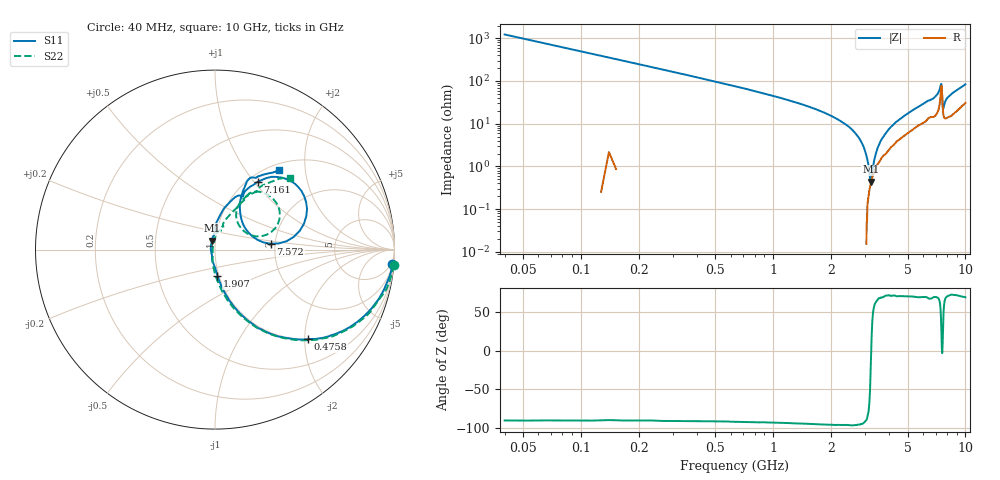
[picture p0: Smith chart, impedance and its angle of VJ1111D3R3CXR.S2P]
! VJ1111D3R3CXR
! DATE 03/04/2022  13:50
! CAPACITORS MOUNTED IN SERIES ON 25 MIL THICK MICROSTRIP SUBSTRATE
# GHz  S  MA  R  50.00
!  FREQ  S11M  S11A  S21M  S21A  S12M  S12A  S22M  S22A
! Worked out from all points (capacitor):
!   801 points, 40 MHz to 10 GHz, reference 50 ohm
!   read as one part in series: C = 3.19 pF near 89.8 MHz
!   lowest |Z| = 436 mohm at 3.215 GHz (marker M1)
!   series resonance near 3.233 GHz, so ESL is about 760 pH
!   S11 on the Smith chart (normalised r, x): 40 MHz: 3, -25; 475.8 MHz: 1.00, -2.06; 1.907 GHz: 0.98, -0.29; 7.161 GHz: 1.11, +1.04; 7.572 GHz: 1.89, +0.14; 10 GHz: 1.11, +1.46
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0.04  0.9893 -4.5  0.08065 85.4  0.08104 85.2  0.9995 -4.9
0.20185  0.9245 -21.8  0.3788 68.4  0.379 68.8  0.9318 -21.9
0.47575  0.7181 -44.1  0.7079 46.9  0.7104 47.1  0.7202 -44.5
0.9613  0.4253 -65.9  0.9241 26.8  0.9278 26.6  0.4189 -66.8
1.7083  0.1882 -81.2  0.9955 13.5  1.001 13.4  0.18 -84.9
1.9075  0.1465 -84.6  0.9998 11.5  1.004 11.3  0.138 -89.4
2.3308  0.07921 -95.5  0.9959 8.0  1.001 7.8  0.06431 -102.2
2.76655  0.02504 -147.3  0.9893 5.3  0.9938 5.2  0.01333 -171.3
2.9035  0.02514 161.6  0.9866 4.8  0.9903 4.6  0.02085 124.7
3.21475  0.05326 108.2  0.9816 3.2  0.9857 3.1  0.0522 93.3
3.36415  0.06719 101.1  0.9768 2.5  0.9813 2.3  0.06608 89.3
3.775  0.1046 85.3  0.9746 0.7  0.9787 0.6  0.1094 76.6
5.02  0.2082 80.1  0.9024 -5.4  0.9067 -5.6  0.2006 68.0
6.6883  0.3417 62.6  0.7999 -12.6  0.8035 -12.7  0.3442 59.6
7.1614  0.4458 57.8  0.7483 -16.6  0.7517 -16.7  0.3958 54.8
7.3606  0.5421 48.0  0.6698 -18.5  0.6729 -18.7  0.4227 46.8
7.4602  0.5793 30.9  0.5674 -14.1  0.5694 -14.3  0.4286 35.7
7.57225  0.3121 6.0  0.6842 5.7  0.6872 5.5  0.2682 16.1
7.6594  0.2154 45.0  0.8166 -2.0  0.8203 -2.2  0.195 49.2
7.89595  0.3464 64.1  0.8118 -11.7  0.8151 -11.8  0.3212 60.9
8.34415  0.4338 64.5  0.7738 -16.4  0.7775 -16.5  0.3985 54.5
10  0.5715 51.1  0.6226 -24.2  0.6256 -24.5  0.578 43.5
